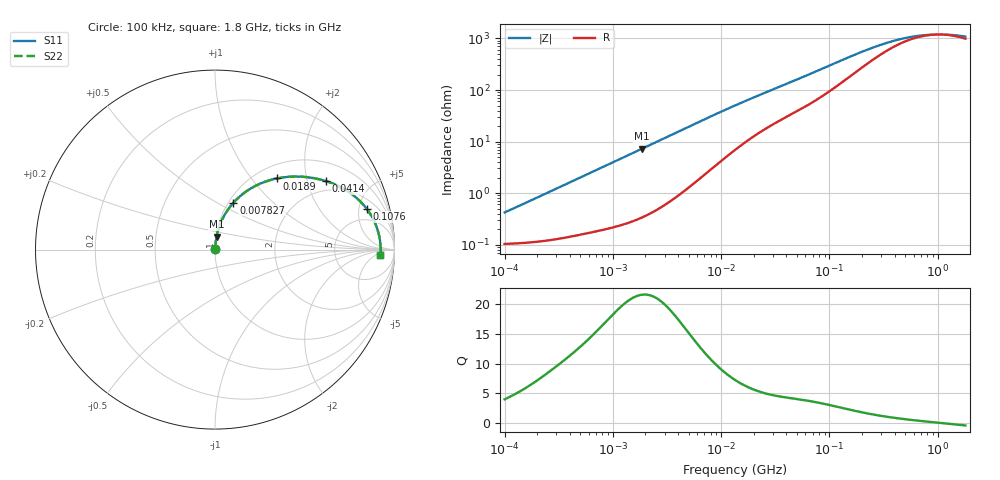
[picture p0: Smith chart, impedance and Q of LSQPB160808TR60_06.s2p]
! LSQPB160808TR60_06  S-PARAMETER MODEL  ( General Type )
! Model Generated by TAIYO YUDEN Corporation (http://www.ty-top.com)
! Version 1.0
! TAIYO YUDEN Control No. 110726NG25SE-FKC
! Copyright(c) 2011 TAIYO YUDEN CO.,LTD. All Rights Reserved.
! Product Description (link to TY-COMPAS)
! https://ds.yuden.co.jp/TYCOMPAS/or/detail?pn=LSQPB160808TR60M06&u=M
! Products Name : Inductors
! Characteristics :
!  Inductance : 0.60 uH , SRF(min) : 630 MHz , DC Resistance(max) : 0.1287 Ohm
!  Rated Current : Saturation :1100 mA , Temp Rise : 940 mA (40 degC)
!  Case Size : 1.6 x 0.8 / 0.063 x 0.031 [mm/inch] , Thickness : 0.8 / 0.031 [mm/inch]
!  (Conditions: Temperature = 25 degC , DC Bias Current/Voltage = 0A / 0V)
! External Node Assignments :
!  1  o---GGG---o  2
! GND o---------o GND
! Frequency Range : 0.1MHz  -  1800MHz  [ 402 STEP ]
# MHz S RI R 50
! Freq[MHz].  S11 Real  S11 Imag  S21 Real  S21 Imag  S12 Real  S12 Imag  S22 Real  S22 Imag
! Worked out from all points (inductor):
!   401 points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, 100 kHz to 1.8 GHz, reference 50 ohm
!   read as one part in series: L = 648 nH near 105 kHz
!   highest Q = 21.6 at 1.845 MHz (marker M1), where L = 622 nH
!   self-resonance near 1.023 GHz
!   S11 on the Smith chart (normalised r, x): 100 kHz: 1.00, +0.01; 7.827 MHz: 1.05, +0.60; 18.9 MHz: 1.23, +1.35; 41.4 MHz: 1.62, +2.63; 107.6 MHz: 3.10, +6.03; 1.8 GHz: 21, -9
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0.1  0.00105 0.00407  0.999 -0.00407  0.999 -0.00407  0.00105 0.00407
0.130924  0.00108 0.00532  0.9989 -0.00532  0.9989 -0.00532  0.00108 0.00532
0.516129  0.00199 0.0205  0.998 -0.0205  0.998 -0.0205  0.00199 0.0205
1.050184  0.0039 0.0411  0.9961 -0.0411  0.9961 -0.0411  0.0039 0.0411
1.844776  0.00845 0.0713  0.9916 -0.0713  0.9916 -0.0713  0.00845 0.0713
2.66389  0.0155 0.1018  0.9845 -0.1018  0.9845 -0.1018  0.0155 0.1018
4.914404  0.0459 0.1793  0.9541 -0.1793  0.9541 -0.1793  0.0459 0.1793
7.827017  0.1028 0.2613  0.8972 -0.2613  0.8972 -0.2613  0.1028 0.2613
10.24746  0.1575 0.3121  0.8425 -0.3121  0.8425 -0.3121  0.1575 0.3121
13.41641  0.2301 0.3574  0.7699 -0.3574  0.7699 -0.3574  0.2301 0.3574
18.90474  0.3433 0.3962  0.6567 -0.3962  0.6567 -0.3962  0.3433 0.3962
27.97575  0.4841 0.4061  0.5159 -0.4061  0.5159 -0.4061  0.4841 0.4061
41.39926  0.6194 0.3813  0.3806 -0.3813  0.3806 -0.3813  0.6194 0.3813
69.24595  0.7651 0.307  0.2349 -0.307  0.2349 -0.307  0.7651 0.307
107.6172  0.8456 0.2268  0.1544 -0.2268  0.1544 -0.2268  0.8456 0.2268
180.0045  0.8935 0.1439  0.1065 -0.1439  0.1065 -0.1439  0.8935 0.1439
259.9299  0.9093 0.0986  0.0907 -0.0986  0.0907 -0.0986  0.9093 0.0986
357.3983  0.9164 0.0681  0.0836 -0.0681  0.0836 -0.0681  0.9164 0.0681
542.0029  0.9209 0.037  0.0791 -0.037  0.0791 -0.037  0.9209 0.037
802.0705  0.9226 0.0134  0.0774 -0.0134  0.0774 -0.0134  0.9226 0.0134
1186.925  0.9229 -0.00816  0.0771 0.00816  0.0771 0.00816  0.9229 -0.00816
1800  0.9219 -0.0326  0.0781 0.0326  0.0781 0.0326  0.9219 -0.0326
